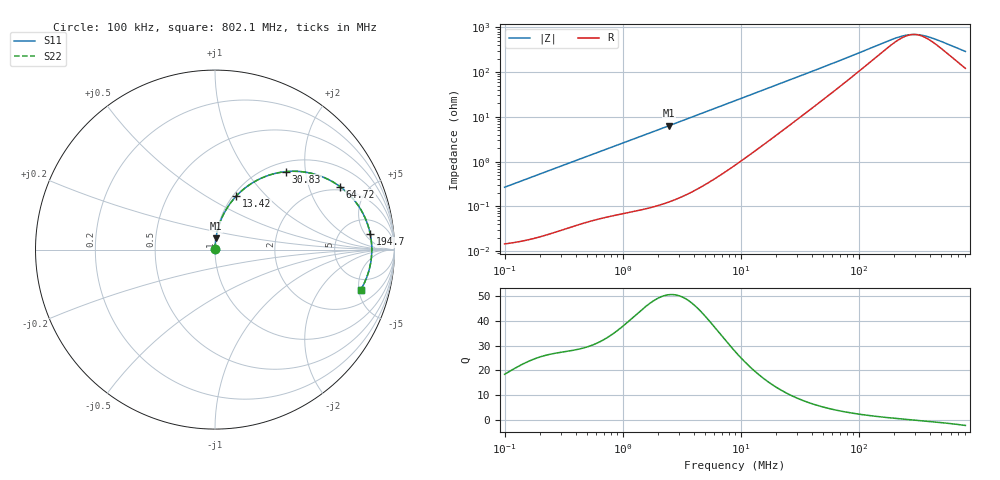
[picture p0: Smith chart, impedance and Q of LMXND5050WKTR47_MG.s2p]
! LMXND5050WKTR47_MG  S-PARAMETER MODEL  ( General Type )
! Model Generated by TAIYO YUDEN Corporation (http://www.ty-top.com)
! Version 1.0
! TAIYO YUDEN Control No. 191023NI43SB-FBB
! Copyright(c) 2019 TAIYO YUDEN CO.,LTD. All Rights Reserved.
! Product Description (link to TY-COMPAS)
! https://ds.yuden.co.jp/TYCOMPAS/or/detail?pn=LMXND5050WKTR47NMG&u=M
! Products Name : Inductors
! Characteristics :
!  Inductance : 0.47 uH , SRF(min) : 230 MHz , DC Resistance(max) : 0.0144 Ohm
!  Rated Current : Saturation :6100 mA , Temp Rise : 5000 mA
!  Case Size : 4.9 x 4.9 / 0.193 x 0.193 [mm/inch] , Thickness : 2 / 0.079 [mm/inch]
!  (Conditions: Temperature = 25 degC , DC Bias Current/Voltage = 0A / 0V)
! External Node Assignments :
!  1  o---GGG---o  2
! GND o---------o GND
! Frequency Range : 0.1MHz  -  802.070463MHz  [ 402 STEP ]
# MHz S RI R 50
! Freq[MHz].  S11 Real  S11 Imag  S21 Real  S21 Imag  S12 Real  S12 Imag  S22 Real  S22 Imag
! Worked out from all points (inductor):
!   401 points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, 100 kHz to 802.1 MHz, reference 50 ohm
!   read as one part in series: L = 425 nH near 104.6 kHz
!   highest Q = 50.5 at 2.487 MHz (marker M1), where L = 407 nH
!   self-resonance near 294 MHz
!   S11 on the Smith chart (normalised r, x): 100 kHz: 1.00, +0.01; 13.42 MHz: 1.04, +0.69; 30.83 MHz: 1.18, +1.57; 64.72 MHz: 1.82, +3.27; 194.7 MHz: 10, +7; 802.1 MHz: 3.42, -5.25
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0.1  0.000152 0.00267  0.9998 -0.00267  0.9998 -0.00267  0.000152 0.00267
0.450771  0.000549 0.0118  0.9995 -0.0118  0.9995 -0.0118  0.000549 0.0118
2.031941  0.00375 0.0518  0.9962 -0.0518  0.9962 -0.0518  0.00375 0.0518
2.487459  0.00528 0.0633  0.9947 -0.0633  0.9947 -0.0633  0.00528 0.0633
4.881709  0.0181 0.1222  0.9819 -0.1222  0.9819 -0.1222  0.0181 0.1222
8.955839  0.0568 0.2141  0.9432 -0.2141  0.9432 -0.2141  0.0568 0.2141
13.42134  0.1176 0.2973  0.8824 -0.2973  0.8824 -0.2973  0.1176 0.2973
20.1134  0.2266 0.3823  0.7734 -0.3823  0.7734 -0.3823  0.2266 0.3823
30.8273  0.3968 0.4346  0.6032 -0.4346  0.6032 -0.4346  0.3968 0.4346
40.37029  0.5169 0.4291  0.4831 -0.4291  0.4831 -0.4291  0.5169 0.4291
50.54372  0.6106 0.4005  0.3894 -0.4005  0.3894 -0.4005  0.6106 0.4005
64.71918  0.6974 0.3504  0.3026 -0.3504  0.3026 -0.3504  0.6974 0.3504
81.0286  0.7584 0.2955  0.2416 -0.2955  0.2416 -0.2955  0.7584 0.2955
103.7538  0.8065 0.2326  0.1935 -0.2326  0.1935 -0.2326  0.8065 0.2326
181.9774  0.8621 0.0999  0.1379 -0.0999  0.1379 -0.0999  0.8621 0.0999
194.67  0.8652 0.0853  0.1348 -0.0853  0.1348 -0.0853  0.8652 0.0853
227.8362  0.8705 0.0522  0.1295 -0.0522  0.1295 -0.0522  0.8705 0.0522
260.727  0.873 0.0244  0.127 -0.0244  0.127 -0.0244  0.873 0.0244
291.7351  0.8737 0.00156  0.1263 -0.00156  0.1263 -0.00156  0.8737 0.00156
333.8503  0.8729 -0.0259  0.1271 0.0259  0.1271 0.0259  0.8729 -0.0259
427.4818  0.8668 -0.0772  0.1332 0.0772  0.1332 0.0772  0.8668 -0.0772
802.0705  0.8124 -0.2231  0.1876 0.2231  0.1876 0.2231  0.8124 -0.2231
